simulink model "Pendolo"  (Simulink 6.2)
settings: Solver=ode45  StartTime=0.0  StopTime=10  RelTol=1e-3
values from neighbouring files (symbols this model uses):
  Cm = 1    [PendParams.m]
  g = 9.81*m/s^2    (= 9.81)    [motoreDC0.m]    (also in PendParams.m = 9.806)
  l = 1.2    [PendParams.m]
  M = 0.25    [PendParams.m]
  q0 = pi/2    (= 1.57079632679)    [PendParams.m]
  w0 = 0    [PendParams.m]
libraries: simulink x1

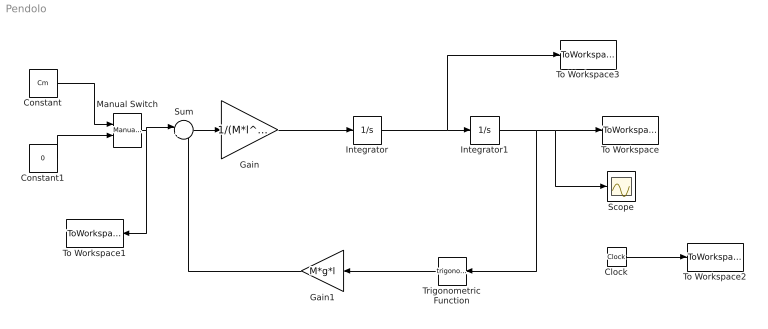
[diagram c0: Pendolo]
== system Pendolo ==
  Clock : Clock
  Constant : Constant  Value=Cm
  Constant1 : Constant  Value=0
  Gain : Gain  Gain=1/(M*l^2)
  Gain1 : Gain  Orientation=left  Gain=M*g*l
  Integrator : Integrator  InitialCondition=w0
  Integrator1 : Integrator  InitialCondition=q0
  Manual Switch : simulink/Signal Routing/Manual Switch  sw=0  action=0
  Scope : Scope
  Sum : Sum  Inputs=|+-
  To Workspace : ToWorkspace  VariableName=q  SampleTime=-1  SaveFormat=Array
  To Workspace1 : ToWorkspace  VariableName=Ci  SampleTime=-1  SaveFormat=Array
  To Workspace2 : ToWorkspace  VariableName=t  SampleTime=-1  SaveFormat=Array
  To Workspace3 : ToWorkspace  VariableName=w  SampleTime=-1  SaveFormat=Array
  Trigonometric Function : Trigonometry  Orientation=left
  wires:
  Gain/1 -> Integrator/1
  Manual Switch/1 -> Sum/1, To Workspace1/1
  Constant1/1 -> Manual Switch/2
  Clock/1 -> To Workspace2/1
  Constant/1 -> Manual Switch/1
  Integrator/1 -> Integrator1/1, To Workspace3/1
  Integrator1/1 -> Trigonometric Function/1, To Workspace/1, Scope/1
  Trigonometric Function/1 -> Gain1/1
  Gain1/1 -> Sum/2
  Sum/1 -> Gain/1
